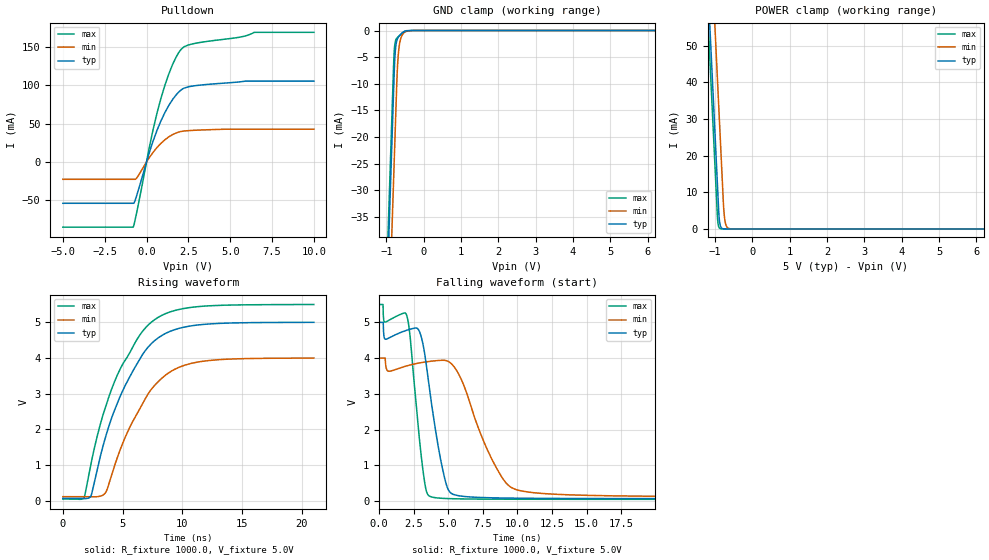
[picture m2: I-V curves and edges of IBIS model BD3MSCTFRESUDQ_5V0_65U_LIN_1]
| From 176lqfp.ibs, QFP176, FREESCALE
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[Model] BD3MSCTFRESUDQ_5V0_65U_LIN_1
Model_type I/O_open_drain
Polarity   Non-Inverting
Enable   Active-High
| var   typ   min   max
C_comp   2.47005pF  2.46575pF  2.47120pF
Vinl = 800.0mV
Vinh = 2.0V
Vmeas = 2.5V
Cref  = 50.0pF
Rref  = 1.0kOhm
Vref  = 5.0V
[Model Spec]
Vinl 800.00000mV 800.00000mV 800.00000mV
Vinh 2.00000V 2.00000V 2.00000V
| variable   typ   min   max
[Temperature Range] 25.0 150.0 -40.0
| variable   typ   min   max
[Voltage Range] 5.0V 4.0V 5.5V
| variable   typ   min   max
[POWER Clamp Reference] 5.0V 4.0V 5.5V
| variable   typ   min   max
[GND Clamp Reference] 0V 0V 0V
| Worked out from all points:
|   slope of the pulldown table from 0 to 0.75 V, typ, clamps not added: 15.8 ohm
|   GND clamp passes 1 mA (typ) near -0.65 V on its own axis
|   POWER clamp passes 1 mA (typ) near -0.86 V on its own axis
|   rising waveform, R_fixture 1000.0, V_fixture 5.0V: 20-80 % time 3.51ns typ, 3.41ns min, 3.6ns max; typ from 0.066 V to 5 V
|   falling waveform, R_fixture 1000.0, V_fixture 5.0V: 20-80 % time 1.16ns typ, 2.39ns min, 791ps max; typ from 5 V to 0.066 V
[POWER Clamp]
-5V       875.6mA    904.4mA    866.6mA
-1.24V    76.57mA    105.4mA    67.61mA
-1.16V    59.57mA    88.38mA    50.61mA
-1.09V    44.69mA    73.5mA     35.73mA
-1.01V    27.69mA    56.5mA     18.73mA
-930mV    10.69mA    39.5mA     2.356mA
-890mV    2.973mA    31mA       332.6uA
-860mV    935uA      24.63mA    82.04uA
-780mV    47.58uA    7.63mA     8.877uA
-750mV    18.44uA    3.369mA    7.12uA
-610mV    3.063uA    76.44uA    3.683uA
10V       0A         0A         0A
[GND Clamp]
-5V       -902.4mA   -919mA     -897.5mA
-1.01V    -54.49mA   -71.14mA   -49.58mA
-810mV    -11.99mA   -28.64mA   -7.082mA
-800mV    -9.863mA   -26.52mA   -5.134mA
-780mV    -5.991mA   -22.27mA   -2.957mA
-750mV    -3.059mA   -15.89mA   -1.788mA
-720mV    -1.885mA   -9.515mA   -1.426mA
-700mV    -1.501mA   -6.433mA   -1.281mA
-680mV    -1.249mA   -4.428mA   -1.146mA
-610mV    -677.8uA   -1.367mA   -660.7uA
-490mV    -100.9uA   -235.7uA   -82.78uA
10V       923.5pA    10.55nA    924.7pA
| variable   typ   min   max
[Pullup Reference] 5.0V 4.0V 5.5V
| variable   typ   min   max
[Pulldown Reference] 0V 0V 0V
[Pullup]
-5V       0A         0A         0A
0V        0A         0A         0A
10V       0A         0A         0A
[Pulldown]
-5V       -53.66mA   -22.48mA   -84.7mA
-790mV    -53.66mA   -22.48mA   -84.33mA
-540mV    -40.34mA   -19.48mA   -60.85mA
390mV     27.06mA    12.51mA    41.86mA
860mV     53.35mA    24.25mA    82.68mA
1.57V     81.59mA    35.75mA    127.3mA
1.92V     90.84mA    38.9mA     142.1mA
2.18V     95.33mA    40.13mA    148.8mA
3.21V     100mA      41.59mA    155.5mA
5.55V     104.2mA    42.7mA     162.3mA
6.44V     105.2mA    42.7mA     168.6mA
10V       105.2mA    42.7mA     168.6mA
[Ramp]
dV/dt_r 2.9602V/3.51078ns 2.33202V/3.41363ns 3.2717V/3.59786ns
dV/dt_f 2.96037V/1.16306ns 2.32973V/2.3891ns 3.27185V/791.17628ps
R_load = 1000.0
| Removed startup time: 0s 0s 0s  .
| Removed end time: 21.01ns.
[Rising Waveform]
R_fixture   = 1000.0
V_fixture   = 5.0V
V_fixture_min = 4.0V
V_fixture_max = 5.5V
0s        65.95mV    112.7mV    46.91mV
1.79ns    59.02mV    112.7mV    94.32mV
2.39ns    165.1mV    112.5mV    1.086V
3.53ns    1.728V     205.6mV    2.578V
5.21ns    3.218V     1.766V     3.928V
6.49ns    4V         2.602V     4.663V
7.55ns    4.446V     3.179V     5.04V
9.19ns    4.773V     3.65V      5.314V
11.24ns   4.923V     3.882V     5.437V
21.03ns   5V         3.999V     5.5V
| Removed startup time: 0s 0s 0s  .
| Removed end time: 27.295ns.
[Falling Waveform]
R_fixture   = 1000.0
V_fixture   = 5.0V
V_fixture_min = 4.0V
V_fixture_max = 5.5V
0s        5V         4V         5.5V
465ps     4.528V     3.898V     5.008V
2.04ns    4.784V     3.786V     5.147V
2.96ns    4.709V     3.867V     1.592V
3.66ns    3.089V     3.908V     133.5mV
4.7ns     711.4mV    3.939V     72.23mV
5.405ns   180.5mV    3.767V     62.82mV
8.11ns    89.88mV    1.205V     51.53mV
9.775ns   79.41mV    337.1mV    49.4mV
27.31ns   66.06mV    117.1mV    46.92mV
